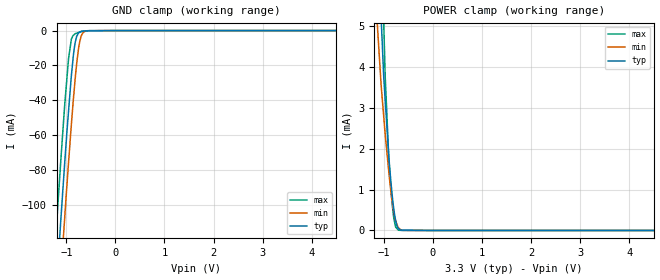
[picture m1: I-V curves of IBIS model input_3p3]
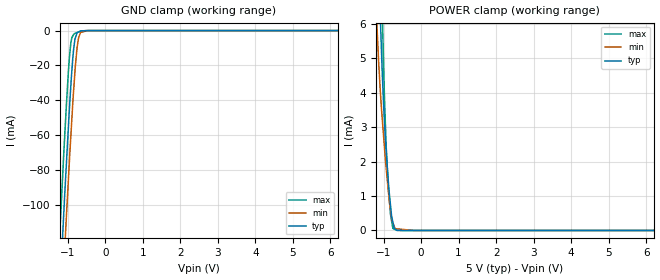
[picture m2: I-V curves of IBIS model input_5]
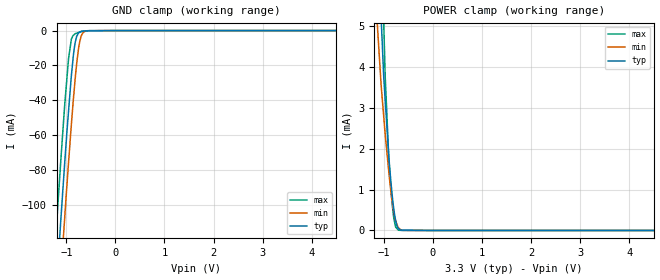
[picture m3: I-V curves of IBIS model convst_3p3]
|Texas Instruments Incorporated
| 16-Bit 1MSPS 0.65 LSB Max INL Precision ADC with Parallel
| Interface and Reference
| Marketing part#   Digital Voltage Range   Package-type   #pins
| ADS8472IBRGZR   2.7 - 5.25V   VQFN   48
| ADS8472IBRGZRG4   2.7 - 5.25V   VQFN   48
| ADS8472IBRGZT   2.7 - 5.25V   VQFN   48
| ADS8472IBRGZTG4   2.7 - 5.25V   VQFN   48
| ADS8472IRGZR   2.7 - 5.25V   VQFN   48
| ADS8472IRGZRG4   2.7 - 5.25V   VQFN   48
| ADS8472IRGZT   2.7 - 5.25V   VQFN   48
| ADS8472IRGZTG4   2.7 - 5.25V   VQFN   48
[IBIS Ver]   3.2
[File name]   ads8472.ibs
|SIMDE Ver   V2.2 - 201009 - RHL4 - Build 424
[File Rev]   1.1
[Date]   03/11/2011
[Source]
| Texas Instruments Incorporated.
| Analog-eLab Design Center, HPA
| 12500 TI Blvd
| Dallas, TX -75243
| e-mail: elab_ibis@list.ti.com
| -Model generated from simulations in TISPICE
[Notes]   Revision History:
| Rev 1.0: 1/21/2011
| - Initial version of the model
| - Model generated from simulations in TISPICE
| - Model matched to SPICE simulation
| - C_comp although listed in numerical order of value are
|   obtained from varying PVT conditions. For PVT conditions for
|   each specific value refer the buffer description under
|   respective [Model]. IBIS model user is responsible for using
|   appropriate C_comp to simulate for Signal Integrity.
| - Model names with a trailing _3p3 contains
|   the model for 3.3V [3.0V and 3.6V]. Model names with trailing _5
|   contains the model for 5.0V [4.75V and 5.25V] operation.
| Rev 1.1: 03/11/2011
| - Updated copyright to 2011
[Disclaimer]
| This model is designed as an aid for customers of Texas Instruments.
| TI and its licensors and suppliers make no warranties, either expressed
| or implied, with respect to this  model, including the warranties of
| merchantability or fitness for a particular purpose. The model is
| provided solely on an "as is" basis. The entire risk as to its quality
| and performance is with the customer.
[Copyright]
 (C) Copyright 2011 Texas Instruments Incorporated.All rights reserved.
|   ADS8472
[Component]   ADS8472
[Manufacturer]   TI
[Package]   |48 VQFN -  RGZ package
|   typ   min   max
R_pkg   0.07524   0.03526   0.09580
L_pkg   1.30242nH   0.84884nH   1.67682nH
C_pkg   0.18098pF   0.15949pF   0.22332pF
[Pin]  signal_name   model_name   R_pin   L_pin   C_pin
1   VBD   POWER   0.08653   1.49778nH  0.18639pF
2   BUS18/_16   input   0.08123   1.39214nH  0.18579pF
3   BYTE   input   0.07444   1.25809nH  0.17595pF
4   _CONVST   convst   0.03526   0.84884nH  0.20541pF
5   _RD   input   0.06511   1.07635nH  0.16537pF
6   _CS   input   0.06340   1.04335nH  0.15949pF
7   VA   POWER   0.06352   1.04565nH  0.15937pF
8   AGND   GND   0.06372   1.04946nH  0.16081pF
9   AGND   GND   0.06603   1.09409nH  0.16410pF
10   VA   POWER   0.07037   1.17840nH  0.16947pF
11   REFM   GND   0.07662   1.30092nH  0.17949pF
12   REFM   GND   0.08201   1.40807nH  0.18102pF
13   REFIN   TERM   0.04479   1.17808nH  0.22332pF
14   REFOUT   TERM   0.08873   1.54172nH  0.19289pF
15   NC   NC   0.08288   1.42449nH  0.18381pF
16   VA   POWER   0.07818   1.33059nH  0.17829pF
17   AGND   GND   0.07484   1.26395nH  0.17388pF
18   IN(+)   TERM   0.07311   1.22895nH  0.17166pF
19   IN(-)   TERM   0.07316   1.22915nH  0.17161pF
20   AGND   GND   0.07497   1.26396nH  0.17392pF
21   VA   POWER   0.07838   1.33059nH  0.17838pF
22   VA   POWER   0.08317   1.42499nH  0.18401pF
23   AGND   GND   0.08905   1.54182nH  0.19073pF
24   AGND   GND   0.08853   1.53187nH  0.18525pF
25   VA   POWER   0.04217   1.02286nH  0.22832pF
26   AGND   GND   0.08115   1.38442nH  0.18975pF
27   AGND   GND   0.03801   0.90449nH  0.21801pF
28   DB17   db   0.07106   1.18459nH  0.17211pF
29   DB16   db   0.06687   1.10246nH  0.16495pF
30   DB15   db   0.06477   1.06155nH  0.16208pF
31   DB14   db   0.06504   1.06675nH  0.16243pF
32   DB13   db   0.06763   1.11736nH  0.16579pF
33   DB12   db   0.07223   1.20769nH  0.17210pF
34   DB11   db   0.07840   1.32969nH  0.17990pF
35   DB10   db   0.08573   1.47572nH  0.19200pF
36   VBD   POWER   0.04364   1.15296nH  0.22385pF
37   BDGND   GND   0.04515   1.17631nH  0.22319pF
38   DB9   db   0.09580   1.67682nH  0.19820pF
39   DB8   db   0.08956   1.55239nH  0.19158pF
40   DB7   db   0.08437   1.44929nH  0.18563pF
41   DB6   db   0.08044   1.37195nH  0.18053pF
42   DB5   db   0.07803   1.32495nH  0.17728pF
43   DB4   db   0.07730   1.31135nH  0.17642pF
44   DB3   db   0.07831   1.33216nH  0.17775pF
45   DB2   db   0.08098   1.38589nH  0.18132pF
46   DB1   db   0.08513   1.46890nH  0.18654pF
47   DB0   db   0.09051   1.57693nH  0.19466pF
48   BUSY   busy   0.09537   1.67458nH  0.19456pF
49   thermal_pad   NC   0.00001   0.00145nH  1.63026pF
[Pin Mapping]  pulldown_ref pullup_ref gnd_clamp_ref power_clamp_ref
1   NC   PWRBUS1
2   GNDBUS1   PWRBUS1
3   GNDBUS1   PWRBUS1
4   GNDBUS1   PWRBUS1
5   GNDBUS1   PWRBUS1
6   GNDBUS1   PWRBUS1
7   NC   PWRBUS2
8   GNDBUS2   NC
9   GNDBUS2   NC
10   NC   PWRBUS2
11   GNDBUS3   NC
12   GNDBUS3   NC
13   GNDBUS2   PWRBUS2
14   GNDBUS2   PWRBUS2
15   NC   NC
16   NC   PWRBUS2
17   GNDBUS2   NC
18   GNDBUS2   PWRBUS2
19   GNDBUS2   PWRBUS2
20   GNDBUS2   NC
21   NC   PWRBUS2
22   NC   PWRBUS2
23   GNDBUS2   NC
24   GNDBUS2   NC
25   NC   PWRBUS2
26   GNDBUS2   NC
27   GNDBUS2   NC
28   GNDBUS1   PWRBUS1
29   GNDBUS1   PWRBUS1
30   GNDBUS1   PWRBUS1
31   GNDBUS1   PWRBUS1
32   GNDBUS1   PWRBUS1
33   GNDBUS1   PWRBUS1
34   GNDBUS1   PWRBUS1
35   GNDBUS1   PWRBUS1
36   NC   PWRBUS1
37   GNDBUS1   NC
38   GNDBUS1   PWRBUS1
39   GNDBUS1   PWRBUS1
40   GNDBUS1   PWRBUS1
41   GNDBUS1   PWRBUS1
42   GNDBUS1   PWRBUS1
43   GNDBUS1   PWRBUS1
44   GNDBUS1   PWRBUS1
45   GNDBUS1   PWRBUS1
46   GNDBUS1   PWRBUS1
47   GNDBUS1   PWRBUS1
48   GNDBUS1   PWRBUS1
49   NC   NC
|   Model Selectors
[Model Selector] input
input_3p3   3.3V digital input
input_5   5.0V digital input
[Model Selector] convst
convst_3p3   3.3V digital input
convst_5   5.0V digital input
[Model Selector] busy
busy_3p3   3.3V digital output
busy_5   5.0V digital output
[Model Selector] db
db_3p3   3.3V 3-state output
db_5   5.0V 3-state output
[Model Selector] TERM
TERM_3p3  3.3V nominal termination
TERM_5   5.0V nominal termination
[Model]  TERM_3p3
Model_type Terminator
C_comp   1.0e-20F  1.0e-20F  1.0e-20F
|   typ   min   max
[Voltage Range]   3.3V   3.0V   3.6V
[POWER Clamp Reference]   3.3V   3.0V   3.6V
[GND Clamp Reference]   0V   0V   0V
|Ambient Temperature   25   85   -40
|Junction Temperature
[Temperature Range]   30   90   -40
[Model]  TERM_5
Model_type Terminator
C_comp   1.0e-20F  1.0e-20F  1.0e-20F
|   typ   min   max
[Voltage Range]   5.0V   4.75V   5.25V
[POWER Clamp Reference]   5.0V   4.75V   5.25V
[GND Clamp Reference]   0V   0V   0V
|Ambient Temperature   25   85   -40
|Junction Temperature
[Temperature Range]   30   90   -40
| Models and submodels in the file (10): input_3p3 (Input), input_5 (Input), convst_3p3 (Input), convst_5 (Input), busy_3p3 (Output), busy_5 (Output), db_3p3 (3-state), db_5 (3-state), TERM_3p3 (Terminator), TERM_5 (Terminator)
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|   input_3p3 Model
[Model]   input_3p3
Model_type   Input
Vinl = 0.8
Vinh = 2.3
|   typ   min   max
|   (nom PVT)   (Fast PVT)   (slow PVT)
|C_comp from frequency method(F=1MHz)
|Average
|C_comp   1.211e-12   1.085e-12   1.349e-12
|C_comp from L-C Tank method(L=1nH)
|Resonant Frequency(Hz)   5.36e9   5.44e9   5.26e9
C_comp   8.826e-13   8.568e-13   9.164e-13
| Where nom  PVT is Nominal Process,  3.3V,  30C
|   Fast PVT is Strong Process,   3.6V,  -40C
|   Slow PVT is Weak Process,   3V,  90C
[Model Spec]
Vinl   0.8   0.8   0.8
Vinh   2.3   2.0   2.6
[Voltage Range]   3.3   3   3.6
|Ambient Temperature   25   85   -40
|Junction Temperature
[Temperature Range]   30   90   -40
[Power Clamp Reference]   3.3   3   3.6
[GND Clamp Reference]   0   0   0
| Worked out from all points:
|   GND clamp passes 1 mA (typ) near -0.73 V on its own axis
|   POWER clamp passes 1 mA (typ) near -0.84 V on its own axis
[GND Clamp]
|   Voltage   I(typ)   I(min)   I(max)
-3.3V     -1.107A    -1.129A    -1.081A
-1.287V   -183.7mA   -214.7mA   -150.2mA
-1.159V   -128.6mA   -159.6mA   -94.06mA
-1.137V   -119mA     -150.1mA   -84.7mA
-1.112V   -108.3mA   -139.8mA   -74.2mA
-1.033V   -75.79mA   -107.1mA   -42.53mA
-954mV    -45.81mA   -75.15mA   -15.73mA
-896.4mV  -25.43mA   -53.39mA   -4.841mA
-810mV    -5.66mA    -24.62mA   -1.68mA
-723mV    -836.2uA   -5.772mA   -858.6uA
-591mV    -229.6uA   -174.9uA   -164.1uA
6.6V      0A         0A         0A
[POWER Clamp]
|   Voltage   I(typ)   I(min)   I(max)
-3.3V     114.3mA    94.22mA    142.1mA
-1.158V   9.058mA    5.513mA    13.01mA
-1.096V   6.558mA    4.315mA    9.552mA
-1.055V   5.194mA    3.537mA    7.319mA
-1.003V   3.763mA    2.793mA    5.098mA
-972mV    3.176mA    2.343mA    3.755mA
-896.4mV  1.759mA    1.395mA    1.692mA
-874.8mV  1.454mA    1.156mA    1.298mA
-795.6mV  513.3uA    430.3uA    288.7uA
-745.8mV  160.8uA    193uA      65.47uA
-702mV    45.96uA    64.11uA    6.738uA
6.6V      0A         0A         0A
|   input_5 Model
[Model]   input_5
Model_type   Input
Vinl = 0.8
Vinh = 4.0
|   typ   min   max
|   (nom PVT)   (Fast PVT)   (slow PVT)
|C_comp from frequency method(F=1MHz)
|Average
|C_comp   1.113e-12   1.007e-12   1.226e-12
|C_comp from L-C Tank method(L=1nH)
|Resonant Frequency(Hz)   5.52e9   5.6e9   5.42e9
C_comp   8.321e-13   8.085e-13   8.631e-13
| Where nom  PVT is Nominal Process,  5V,  30C
|   Fast PVT is Strong Process,   5.25V,  -40C
|   Slow PVT is Weak Process,   4.75V,  90C
[Model Spec]
Vinl   0.8   0.8   0.8
Vinh   4.0   3.75   4.25
[Voltage Range]   5   4.75   5.25
|Ambient Temperature   25   85   -40
|Junction Temperature
[Temperature Range]   30   90   -40
[Power Clamp Reference]   5   4.75   5.25
[GND Clamp Reference]   0   0   0
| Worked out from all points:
|   GND clamp passes 1 mA (typ) near -0.73 V on its own axis
|   POWER clamp passes 1 mA (typ) near -0.84 V on its own axis
[GND Clamp]
|   Voltage   I(typ)   I(min)   I(max)
-5V       -1.898A    -1.916A    -1.876A
-1.306V   -192.2mA   -223.1mA   -158.4mA
-1.108V   -106.7mA   -138mA     -72.38mA
-1.08V    -94.88mA   -126.2mA   -61.18mA
-1.04V    -78.88mA   -109.4mA   -44.94mA
-950.3mV  -43.75mA   -73.69mA   -14.72mA
-913.5mV  -31.06mA   -60mA      -6.967mA
-840mV    -10.48mA   -34.09mA   -2.163mA
-745.8mV  -1.183mA   -9.257mA   -1.102mA
-707.7mV  -789.6uA   -4.052mA   -791.6uA
-640mV    -158.4uA   -951.7uA   -242uA
10V       0A         0A         0A
[POWER Clamp]
|   Voltage   I(typ)   I(min)   I(max)
-5V       200.2mA    168.8mA    246.3mA
-1.178V   10.06mA    6.005mA    13.91mA
-1.08V    6.013mA    3.952mA    8.603mA
-1.064V   5.51mA     3.682mA    7.807mA
-1.035V   4.599mA    3.255mA    6.396mA
-990mV    3.456mA    2.619mA    4.468mA
-929.3mV  2.319mA    1.811mA    2.435mA
-876.8mV  1.492mA    1.196mA    1.331mA
-813.7mV  723.3uA    596.6uA    459.2uA
-750.8mV  240uA      226.2uA    58.49uA
-640.5mV  4.904uA    46.48uA    457nA
10V       0A         0A         0A
|   convst_3p3 Model
[Model]   convst_3p3
Model_type   Input
Vinl = 0.8
Vinh = 2.3
|   typ   min   max
|   (nom PVT)   (Fast PVT)   (slow PVT)
|C_comp from frequency method(F=1MHz)
|Average
|C_comp   1.462e-12   1.335e-12   1.599e-12
|C_comp from L-C Tank method(L=1nH)
|Resonant Frequency(Hz)   4.68e9   4.75e9   4.61e9
C_comp   1.158e-12   1.124e-12   1.193e-12
| Where nom  PVT is Nominal Process,  3.3V,  30C
|   Fast PVT is Strong Process,   3.6V,  -40C
|   Slow PVT is Weak Process,   3V,  90C
[Model Spec]
Vinl   0.8   0.8   0.8
Vinh   2.3   2.0   2.6
[Voltage Range]   3.3   3   3.6
|Ambient Temperature   25   85   -40
|Junction Temperature
[Temperature Range]   30   90   -40
[Power Clamp Reference]   3.3   3   3.6
[GND Clamp Reference]   0   0   0
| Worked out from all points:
|   GND clamp passes 1 mA (typ) near -0.73 V on its own axis
|   POWER clamp passes 1 mA (typ) near -0.84 V on its own axis
[GND Clamp]
|   Voltage   I(typ)   I(min)   I(max)
-3.3V     -1.107A    -1.129A    -1.081A
-1.287V   -183.7mA   -214.7mA   -150.2mA
-1.159V   -128.6mA   -159.6mA   -94.06mA
-1.137V   -119mA     -150.1mA   -84.7mA
-1.112V   -108.3mA   -139.8mA   -74.2mA
-1.033V   -75.79mA   -107.1mA   -42.53mA
-954mV    -45.81mA   -75.15mA   -15.73mA
-896.4mV  -25.43mA   -53.39mA   -4.841mA
-810mV    -5.66mA    -24.62mA   -1.68mA
-723mV    -836.2uA   -5.772mA   -858.6uA
-591mV    -229.6uA   -174.9uA   -164.1uA
6.6V      0A         0A         0A
[POWER Clamp]
|   Voltage   I(typ)   I(min)   I(max)
-3.3V     114.3mA    94.22mA    142.1mA
-1.158V   9.058mA    5.513mA    13.01mA
-1.096V   6.558mA    4.315mA    9.552mA
-1.055V   5.194mA    3.537mA    7.319mA
-1.003V   3.763mA    2.793mA    5.098mA
-972mV    3.176mA    2.343mA    3.755mA
-896.4mV  1.759mA    1.395mA    1.692mA
-874.8mV  1.454mA    1.156mA    1.298mA
-795.6mV  513.3uA    430.3uA    288.7uA
-745.8mV  160.8uA    193uA      65.47uA
-702mV    45.96uA    64.11uA    6.738uA
6.6V      0A         0A         0A
